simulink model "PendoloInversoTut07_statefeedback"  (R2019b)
settings: Solver=ode4  StartTime=0  StopTime=120  FixedStep=0.0001  MaxStep=0.02  RelTol=1e-3  AbsTol=1e-6
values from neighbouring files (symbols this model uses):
  A = [0      1              0           0    [PendInvCarrello_Svolgimento.m]
  B = [ 0; (I+m*l^2)/p; 0; m*l/p]    [PendInvCarrello_Svolgimento.m]
  C = [1 0 0 0; 0 0 1 0]    [PendInvCarrello_Svolgimento.m]
  K = Kbar*inv(T)    [PendInvCarrello_Svolgimento.m]
  mu = dcgain(Gry)    [PendInvCarrello_Svolgimento.m]
  Tc = 0.02    [PendInvCarrello_Svolgimento.m]
undefined symbols (not defined in the file or in its folder): Reference

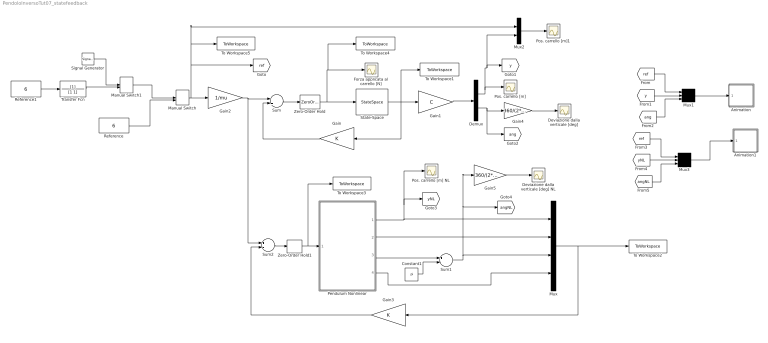
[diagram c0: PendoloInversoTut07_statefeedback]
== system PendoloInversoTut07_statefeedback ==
  Animation : Subsystem  mask(Pendulum plot){RefBlock=Reference}
      mask prompts: RefBlock "DC reference signal block name:"
      mask help: Pendulum plot
  Animation1 : Subsystem  mask(Pendulum plot){RefBlock=Reference}
      mask prompts: RefBlock "DC reference signal block name:"
      mask help: Pendulum plot
  Constant1 : Constant  Value=pi
  Demux : Demux  Outputs=2
  Deviazione dalla verticale [deg] NL : Scope
  Deviazione dalla verticale [deg] : Scope
  Forza applicata al carrello [N] : Scope
  Gain : Gain  Gain=K  Multiplication=Matrix(K*u)
  Gain1 : Gain  Gain=C  Multiplication=Matrix(K*u)
  Gain2 : Gain  Gain=1/mu
  Gain3 : Gain  Gain=K  Multiplication=Matrix(K*u)
  Gain4 : Gain  Gain=360/(2*pi)
  Gain5 : Gain  Gain=360/(2*pi)
  Manual Switch : ManualSwitch  CurrentSetting=0
  Manual Switch1 : ManualSwitch
  Mux : Mux
  Mux1 : Mux  Inputs=3
  Mux2 : Mux  Inputs=2
  Mux3 : Mux  Inputs=3
  Pendulum Nonlinear : Subsystem
  Pos. carrello [m] : Scope
  Pos. carrello [m] NL : Scope
  Pos. carrello [m]1 : Scope
  Reference : Constant  Value=6  VectorParams1D=off
  Reference1 : Constant  Value=6  VectorParams1D=off
  Signal Generator : SignalGenerator  Amplitude=6  Frequency=0.04  Units=rad/sec
  State-Space : StateSpace  A=A  B=B  C=eye(4)  D=zeros(4,1)  InitialCondition=0
  Sum : Sum  Inputs=+-
  Sum1 : Sum  Inputs=+-
  Sum2 : Sum  Inputs=+-
  To Workspace1 : ToWorkspace  VariableName=x  SaveFormat=Timeseries  SampleTime=-1
  To Workspace2 : ToWorkspace  VariableName=x_NL  SaveFormat=Timeseries  SampleTime=-1
  To Workspace3 : ToWorkspace  VariableName=F_NL  SaveFormat=Timeseries  SampleTime=-1
  To Workspace4 : ToWorkspace  VariableName=F  SaveFormat=Timeseries  SampleTime=-1
  To Workspace5 : ToWorkspace  VariableName=Ref  SaveFormat=Timeseries  SampleTime=-1
  Transfer Fcn : TransferFcn  Denominator=[1 1]
  Zero-Order Hold : ZeroOrderHold  SampleTime=Tc
  Zero-Order Hold1 : ZeroOrderHold  SampleTime=Tc
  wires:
  Mux1/1 -> Animation/1(in_1)
  Sum/1 -> Zero-Order Hold/1
  Zero-Order Hold/1 -> To Workspace4/1, Forza applicata al carrello [N]/1, State-Space/1
  Demux/1 -> Mux2/2, [y], Pos. carrello [m]/1
  Gain/1 -> Sum/2
  State-Space/1 -> Gain1/1, To Workspace1/1, Gain/1
  Demux/2 -> [ang], Gain4/1
  Gain1/1 -> Demux/1
  Gain2/1 -> Sum2/1, Sum/1
  [y] -> Mux1/2
  Constant1/1 -> Sum1/2
  [ang] -> Mux1/3
  Pendulum Nonlinear/1(CarrPos) -> [yNL], Pos. carrello [m] NL/1, Mux/1
  Pendulum Nonlinear/2(CarrVel) -> Mux/2
  Pendulum Nonlinear/3(Angle) -> Sum1/1
  Sum1/1 -> Mux/3, Gain5/1, [angNL]
  Pendulum Nonlinear/4(AngleDer) -> Mux/4
  Mux/1 -> Gain3/1, To Workspace2/1
  Gain3/1 -> Sum2/2
  Sum2/1 -> Zero-Order Hold1/1
  Zero-Order Hold1/1 -> To Workspace3/1, Pendulum Nonlinear/1(F)
  Manual Switch/1 -> Mux2/1, To Workspace5/1, [ref], Gain2/1
  Reference/1 -> Manual Switch/2
  [ref] -> Mux1/1
  Gain4/1 -> Deviazione dalla verticale [deg]/1
  Gain5/1 -> Deviazione dalla verticale [deg] NL/1
  Reference1/1 -> Transfer Fcn/1
  Transfer Fcn/1 -> Manual Switch1/2
  Signal Generator/1 -> Manual Switch1/1
  Manual Switch1/1 -> Manual Switch/1
  Mux2/1 -> Pos. carrello [m]1/1
  [ref] -> Mux3/1
  [angNL] -> Mux3/3
  Mux3/1 -> Animation1/1(in_1)
  [yNL] -> Mux3/2

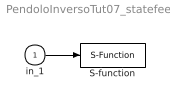
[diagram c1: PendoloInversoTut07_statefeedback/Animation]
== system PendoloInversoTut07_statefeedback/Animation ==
  in_1 : Inport
  S-function : S-Function  FunctionName=pendan_file  Parameters=RefBlock  SFunctionDeploymentMode=off  EnableBusSupport=off
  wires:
  in_1/1 -> S-function/1

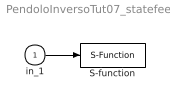
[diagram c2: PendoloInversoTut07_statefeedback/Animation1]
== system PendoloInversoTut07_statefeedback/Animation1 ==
  in_1 : Inport
  S-function : S-Function  FunctionName=pendan_fileNL  Parameters=RefBlock  SFunctionDeploymentMode=off  EnableBusSupport=off
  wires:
  in_1/1 -> S-function/1

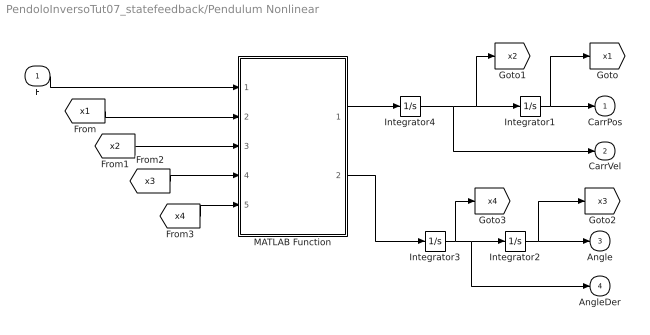
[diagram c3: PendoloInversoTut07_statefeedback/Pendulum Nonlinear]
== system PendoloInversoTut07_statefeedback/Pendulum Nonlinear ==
  F : Inport
  Integrator1 : Integrator
  Integrator2 : Integrator  InitialCondition=pi
  Integrator3 : Integrator
  Integrator4 : Integrator
  MATLAB Function : MATLAB Function  TreatAsAtomicUnit=on
  CarrPos : Outport  InitialOutput=0  VectorParamsAs1DForOutWhenUnconnected=off
  CarrVel : Outport  Port=2  InitialOutput=0  VectorParamsAs1DForOutWhenUnconnected=off
  Angle : Outport  Port=3  InitialOutput=0  VectorParamsAs1DForOutWhenUnconnected=off
  AngleDer : Outport  Port=4  InitialOutput=0  VectorParamsAs1DForOutWhenUnconnected=off
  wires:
  Integrator1/1 -> [x1], CarrPos/1
  MATLAB Function/2(teta_ddot) -> Integrator3/1
  MATLAB Function/1(yddot) -> Integrator4/1
  Integrator4/1 -> CarrVel/1, [x2], Integrator1/1
  F/1 -> MATLAB Function/1(F)
  Integrator3/1 -> [x4], AngleDer/1, Integrator2/1
  Integrator2/1 -> [x3], Angle/1
  [x1] -> MATLAB Function/2(x1)
  [x2] -> MATLAB Function/3(x2)
  [x3] -> MATLAB Function/4(x3)
  [x4] -> MATLAB Function/5(x4)

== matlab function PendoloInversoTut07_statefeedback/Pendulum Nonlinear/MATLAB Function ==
function [yddot,teta_ddot] = fcn(F,x1,x2,x3,x4)

M = 0.5;
m = 0.2;
b = 0.1;
I = 0.006;
l = 0.3;
g = 9.8;

Delta=(M+m)*(I+m*l^2)-m^2*l^2*cos(x3)^2;

yddot = -b*(I+m*l^2)*x2/Delta+m*l*x4^2*sin(x3)/Delta+m^2*g*l^2*sin(x3)*cos(x3)/Delta+(I+m*l^2)*F/Delta;

teta_ddot=m*l*b*cos(x3)*x2/Delta-m^2*l^2*x4^2*sin(x3)*cos(x3)/Delta-(M+m)*m*g*l*sin(x3)/Delta-m*l*cos(x3)*F/Delta;
